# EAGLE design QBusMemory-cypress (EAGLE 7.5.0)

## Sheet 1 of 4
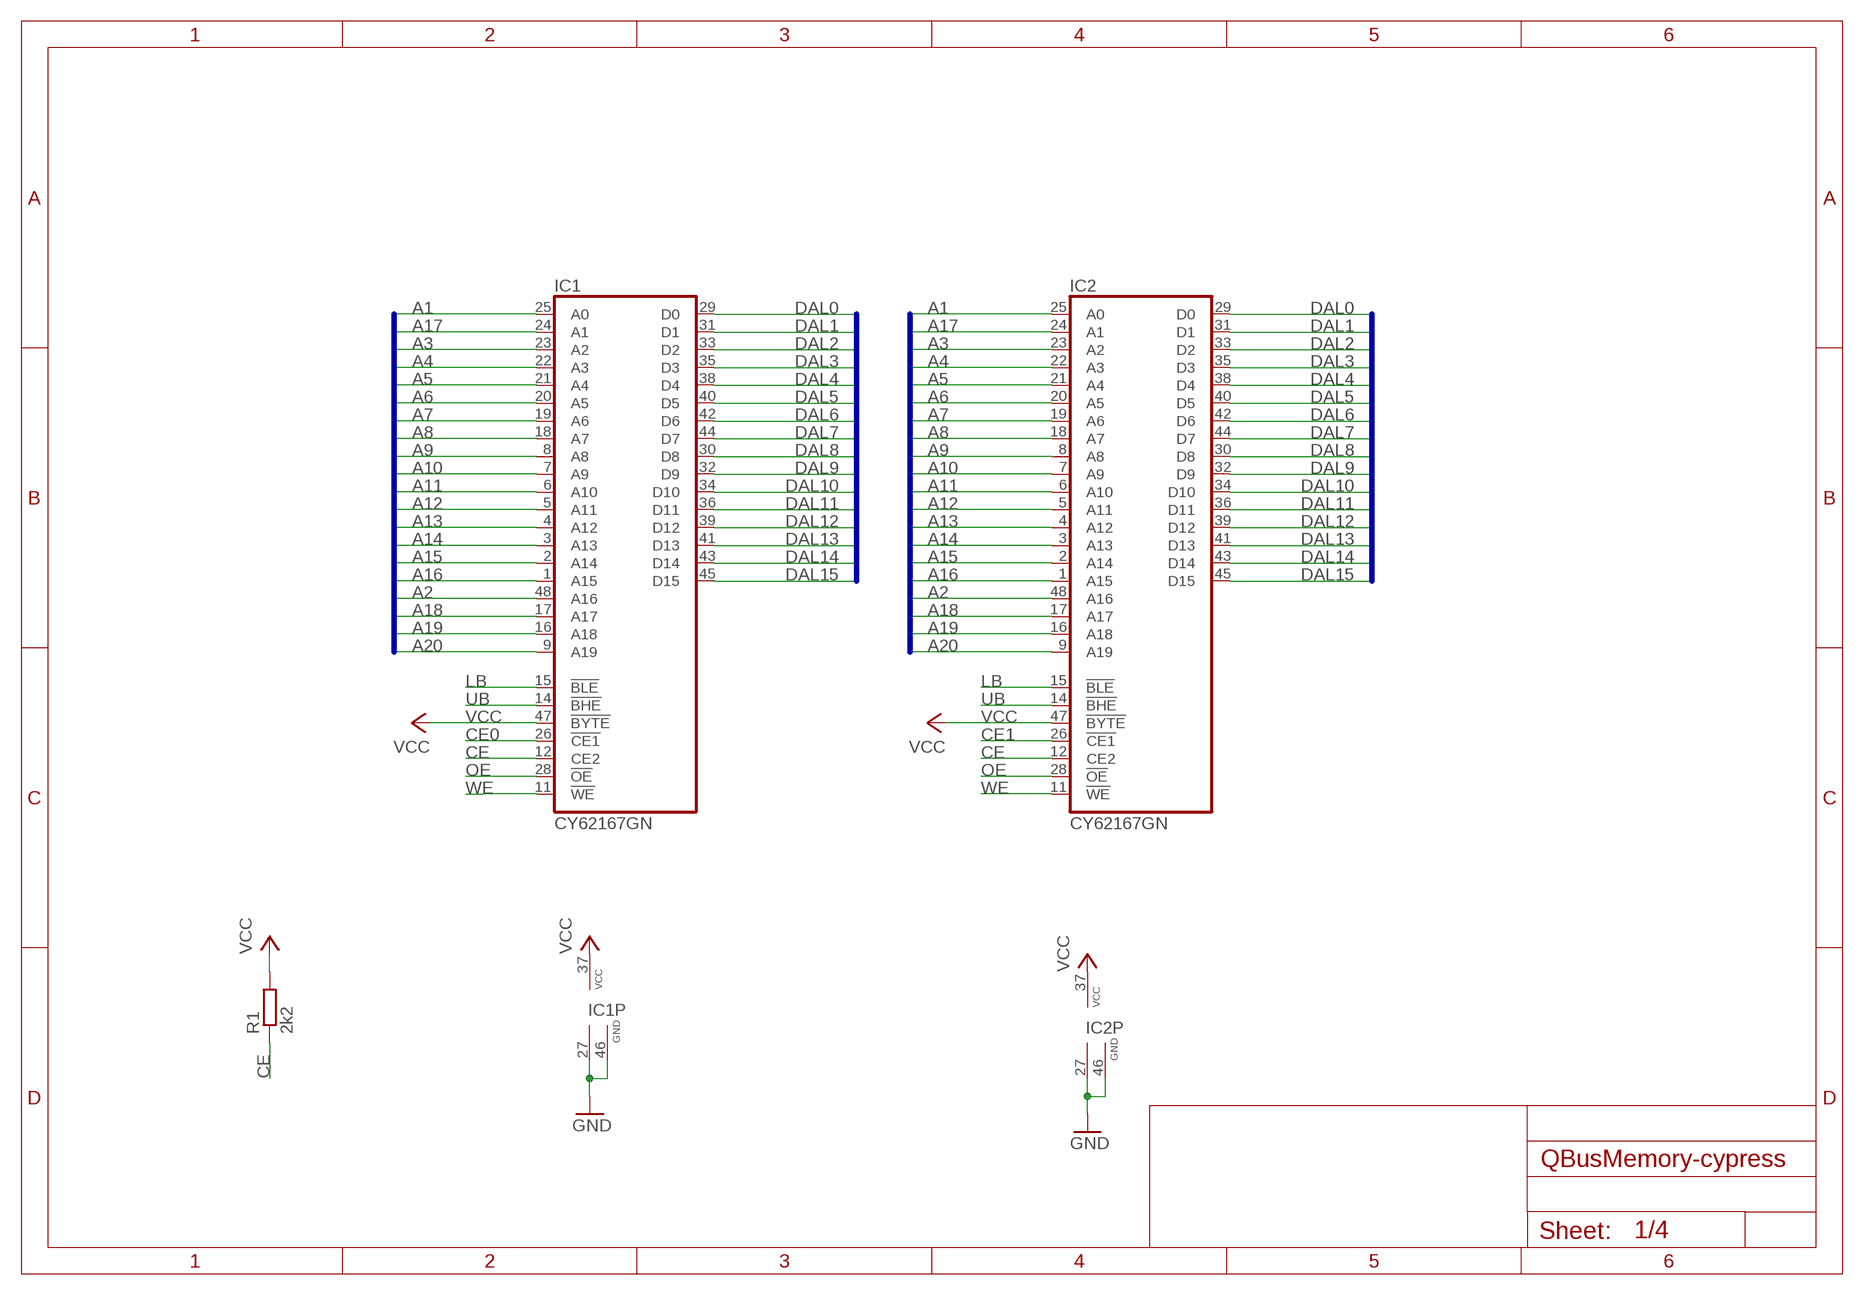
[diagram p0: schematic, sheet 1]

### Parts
IC1  CY62167GN  CY62167  [TSOP48]
IC2  CY62167GN  CY62167  [TSOP48]
R1  2k2  R-EU_R0805  [R0805]

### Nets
A1: IC1.25(A0) IC2.25(A0) ; also sheet 4
A2: IC1.48(A16) IC2.48(A16) ; also sheet 4
A3: IC1.23(A2) IC2.23(A2) ; also sheet 4
A4: IC1.22(A3) IC2.22(A3) ; also sheet 4
A5: IC1.21(A4) IC2.21(A4) ; also sheet 3
A6: IC1.20(A5) IC2.20(A5) ; also sheet 3
A7: IC1.19(A6) IC2.19(A6) ; also sheet 3
A8: IC1.18(A7) IC2.18(A7) ; also sheet 3
A9: IC1.8(A8) IC2.8(A8) ; also sheet 3
A10: IC1.7(A9) IC2.7(A9) ; also sheet 3
A11: IC1.6(A10) IC2.6(A10) ; also sheet 3
A12: IC1.5(A11) IC2.5(A11) ; also sheet 3
A13: IC1.4(A12) IC2.4(A12) ; also sheet 3
A14: IC1.3(A13) IC2.3(A13) ; also sheet 3
A15: IC1.2(A14) IC2.2(A14) ; also sheet 3
A16: IC1.1(A15) IC2.1(A15) ; also sheet 3
A17: IC1.24(A1) IC2.24(A1) ; also sheet 3
A18: IC1.17(A17) IC2.17(A17) ; also sheet 3
A19: IC1.16(A18) IC2.16(A18) ; also sheet 3
A20: IC1.9(A19) IC2.9(A19) ; also sheet 3
CE: IC1.12(CE2) IC2.12(CE2) R1.1
CE0: IC1.26(!CE1) ; also sheet 4
CE1: IC2.26(!CE1) ; also sheet 4
DAL0: IC1.29(D0) IC2.29(D0) ; also sheet 3,4
DAL1: IC1.31(D1) IC2.31(D1) ; also sheet 3,4
DAL2: IC1.33(D2) IC2.33(D2) ; also sheet 3,4
DAL3: IC1.35(D3) IC2.35(D3) ; also sheet 3,4
DAL4: IC1.38(D4) IC2.38(D4) ; also sheet 3,4
DAL5: IC1.40(D5) IC2.40(D5) ; also sheet 3
DAL6: IC1.42(D6) IC2.42(D6) ; also sheet 3
DAL7: IC1.44(D7) IC2.44(D7) ; also sheet 3
DAL8: IC1.30(D8) IC2.30(D8) ; also sheet 3
DAL9: IC1.32(D9) IC2.32(D9) ; also sheet 3
DAL10: IC1.34(D10) IC2.34(D10) ; also sheet 3
DAL11: IC1.36(D11) IC2.36(D11) ; also sheet 3
DAL12: IC1.39(D12) IC2.39(D12) ; also sheet 3
DAL13: IC1.41(D13) IC2.41(D13) ; also sheet 3
DAL14: IC1.43(D14) IC2.43(D14) ; also sheet 3
DAL15: IC1.45(D15) IC2.45(D15) ; also sheet 3
GND: IC1.27(GND) IC1.46(GND) IC2.27(GND) IC2.46(GND) ; also sheet 2,3,4
LB: IC1.15(!BLE) IC2.15(!BLE) ; also sheet 4
OE: IC1.28(!OE) IC2.28(!OE) ; also sheet 4
UB: IC1.14(!BHE) IC2.14(!BHE) ; also sheet 4
VCC: IC1.37(VCC) IC1.47(!BYTE) IC2.37(VCC) IC2.47(!BYTE) R1.2 ; also sheet 2,3,4
WE: IC1.11(!WE) IC2.11(!WE) ; also sheet 4
Unconnected: IC1.10(NC) IC1.13(NC) IC2.10(NC) IC2.13(NC)

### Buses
A[0..21]
DAL[0..21]

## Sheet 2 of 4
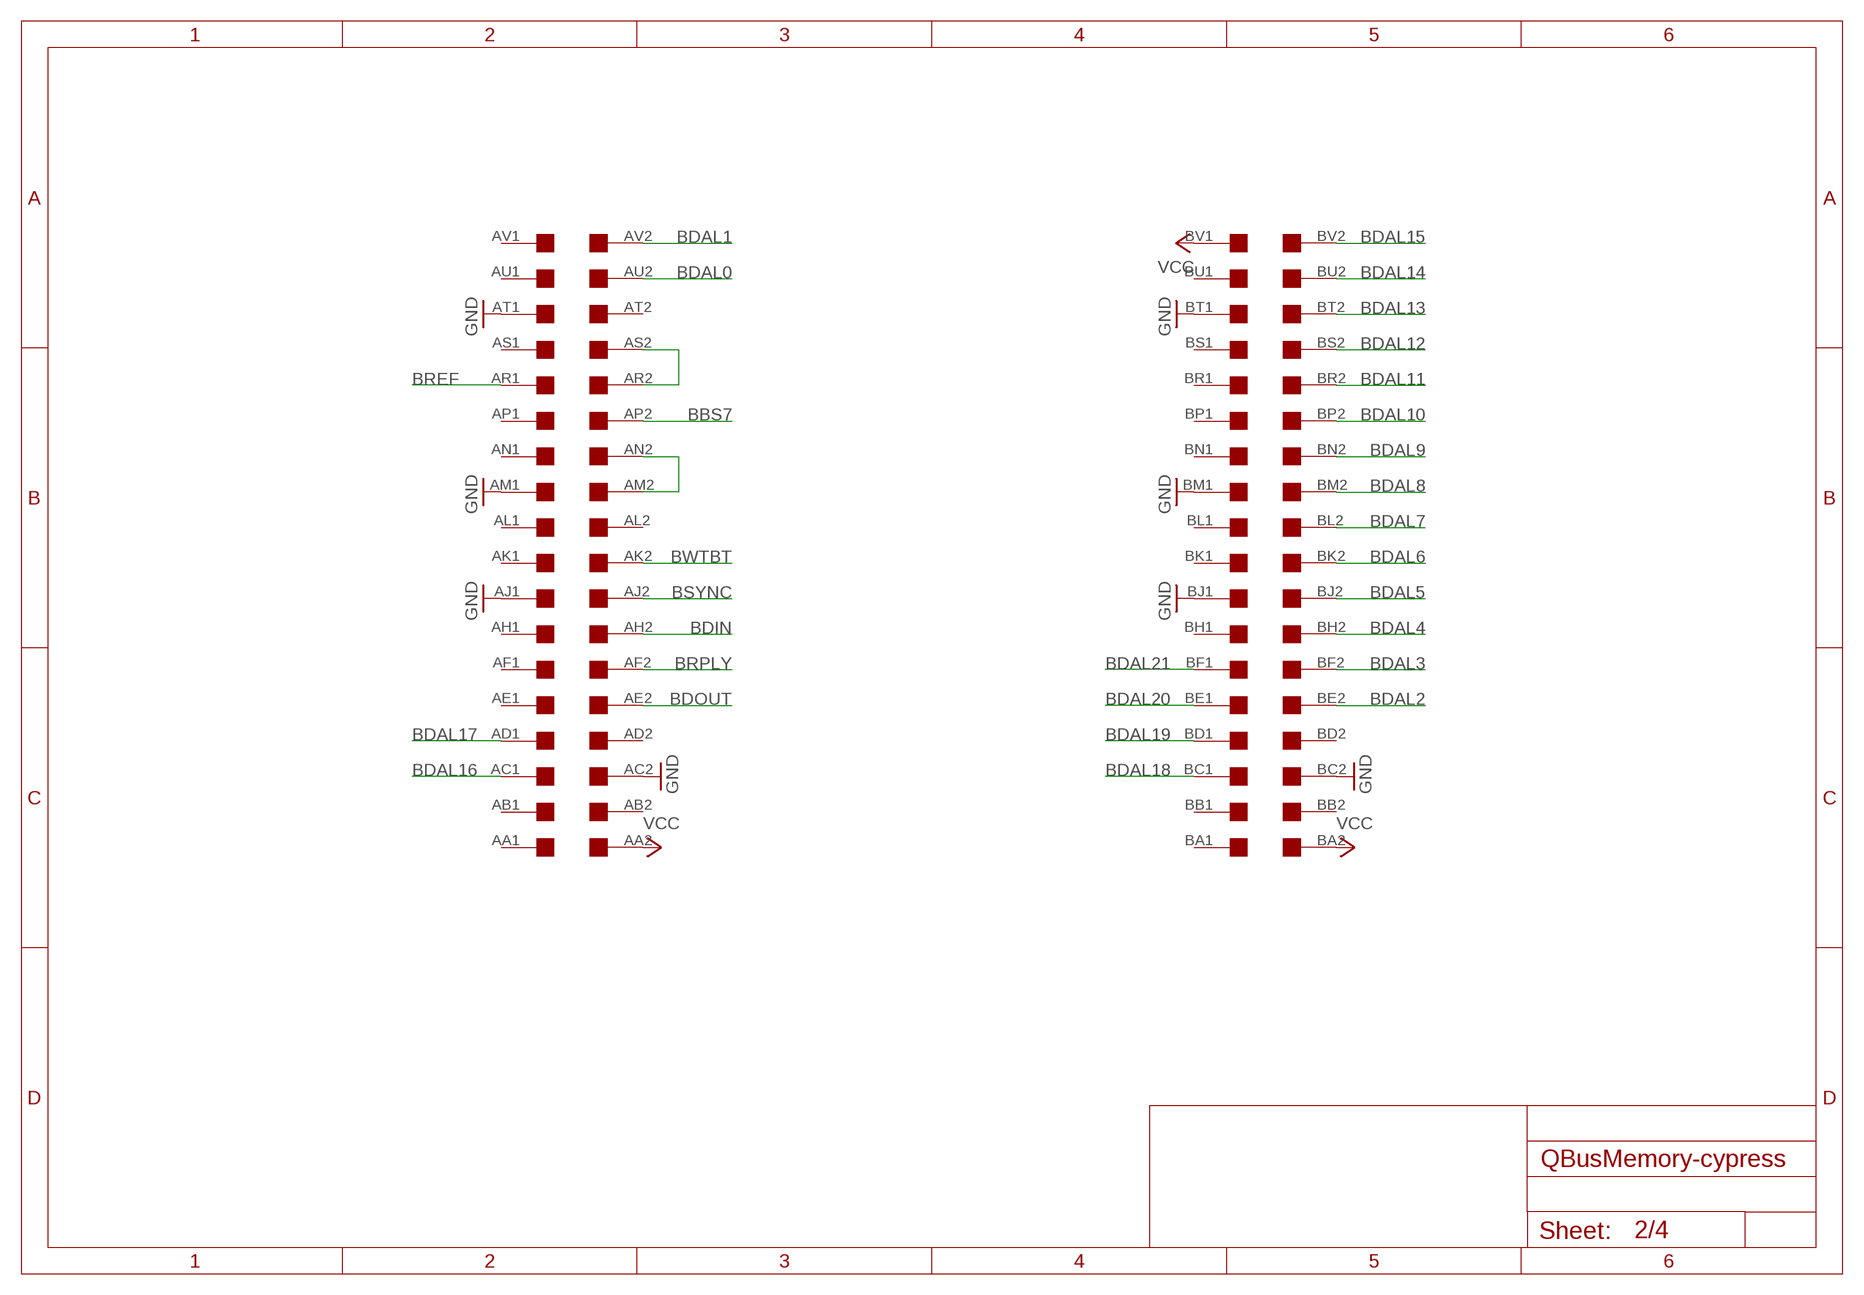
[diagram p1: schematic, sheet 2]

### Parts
U$1  DOUBLE  [EDGE-CON4]

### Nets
BBS7: U$1.AP2 ; also sheet 3
BDAL0: U$1.AU2 ; also sheet 3
BDAL1: U$1.AV2 ; also sheet 3
BDAL2: U$1.BE2 ; also sheet 3
BDAL3: U$1.BF2 ; also sheet 3
BDAL4: U$1.BH2 ; also sheet 3
BDAL5: U$1.BJ2 ; also sheet 3
BDAL6: U$1.BK2 ; also sheet 3
BDAL7: U$1.BL2 ; also sheet 3
BDAL8: U$1.BM2 ; also sheet 3
BDAL9: U$1.BN2 ; also sheet 3
BDAL10: U$1.BP2 ; also sheet 3
BDAL11: U$1.BR2 ; also sheet 3
BDAL12: U$1.BS2 ; also sheet 3
BDAL13: U$1.BT2 ; also sheet 3
BDAL14: U$1.BU2 ; also sheet 3
BDAL15: U$1.BV2 ; also sheet 3
BDAL16: U$1.AC1 ; also sheet 3
BDAL17: U$1.AD1 ; also sheet 3
BDAL18: U$1.BC1 ; also sheet 3
BDAL19: U$1.BD1 ; also sheet 3
BDAL20: U$1.BE1 ; also sheet 3
BDAL21: U$1.BF1 ; also sheet 3
BDIN: U$1.AH2 ; also sheet 3
BDOUT: U$1.AE2 ; also sheet 3
BREF: U$1.AR1 ; also sheet 3
BRPLY: U$1.AF2 ; also sheet 3
BSYNC: U$1.AJ2 ; also sheet 3
BWTBT: U$1.AK2 ; also sheet 3
GND: U$1.AC2 U$1.AJ1 U$1.AM1 U$1.AT1 U$1.BC2 U$1.BJ1 U$1.BM1 U$1.BT1 ; also sheet 1,3,4
N$1: U$1.AR2 U$1.AS2
N$2: U$1.AM2 U$1.AN2
VCC: U$1.AA2 U$1.BA2 U$1.BV1 ; also sheet 1,3,4
Unconnected: U$1.AA1 U$1.AB1 U$1.AB2 U$1.AD2 U$1.AE1 U$1.AF1 U$1.AH1 U$1.AK1 U$1.AL1 U$1.AL2 U$1.AN1 U$1.AP1 U$1.AS1 U$1.AT2 U$1.AU1 U$1.AV1 U$1.BA1 U$1.BB1 U$1.BB2 U$1.BD2 U$1.BH1 U$1.BK1 U$1.BL1 U$1.BN1 U$1.BP1 U$1.BR1 U$1.BS1 U$1.BU1

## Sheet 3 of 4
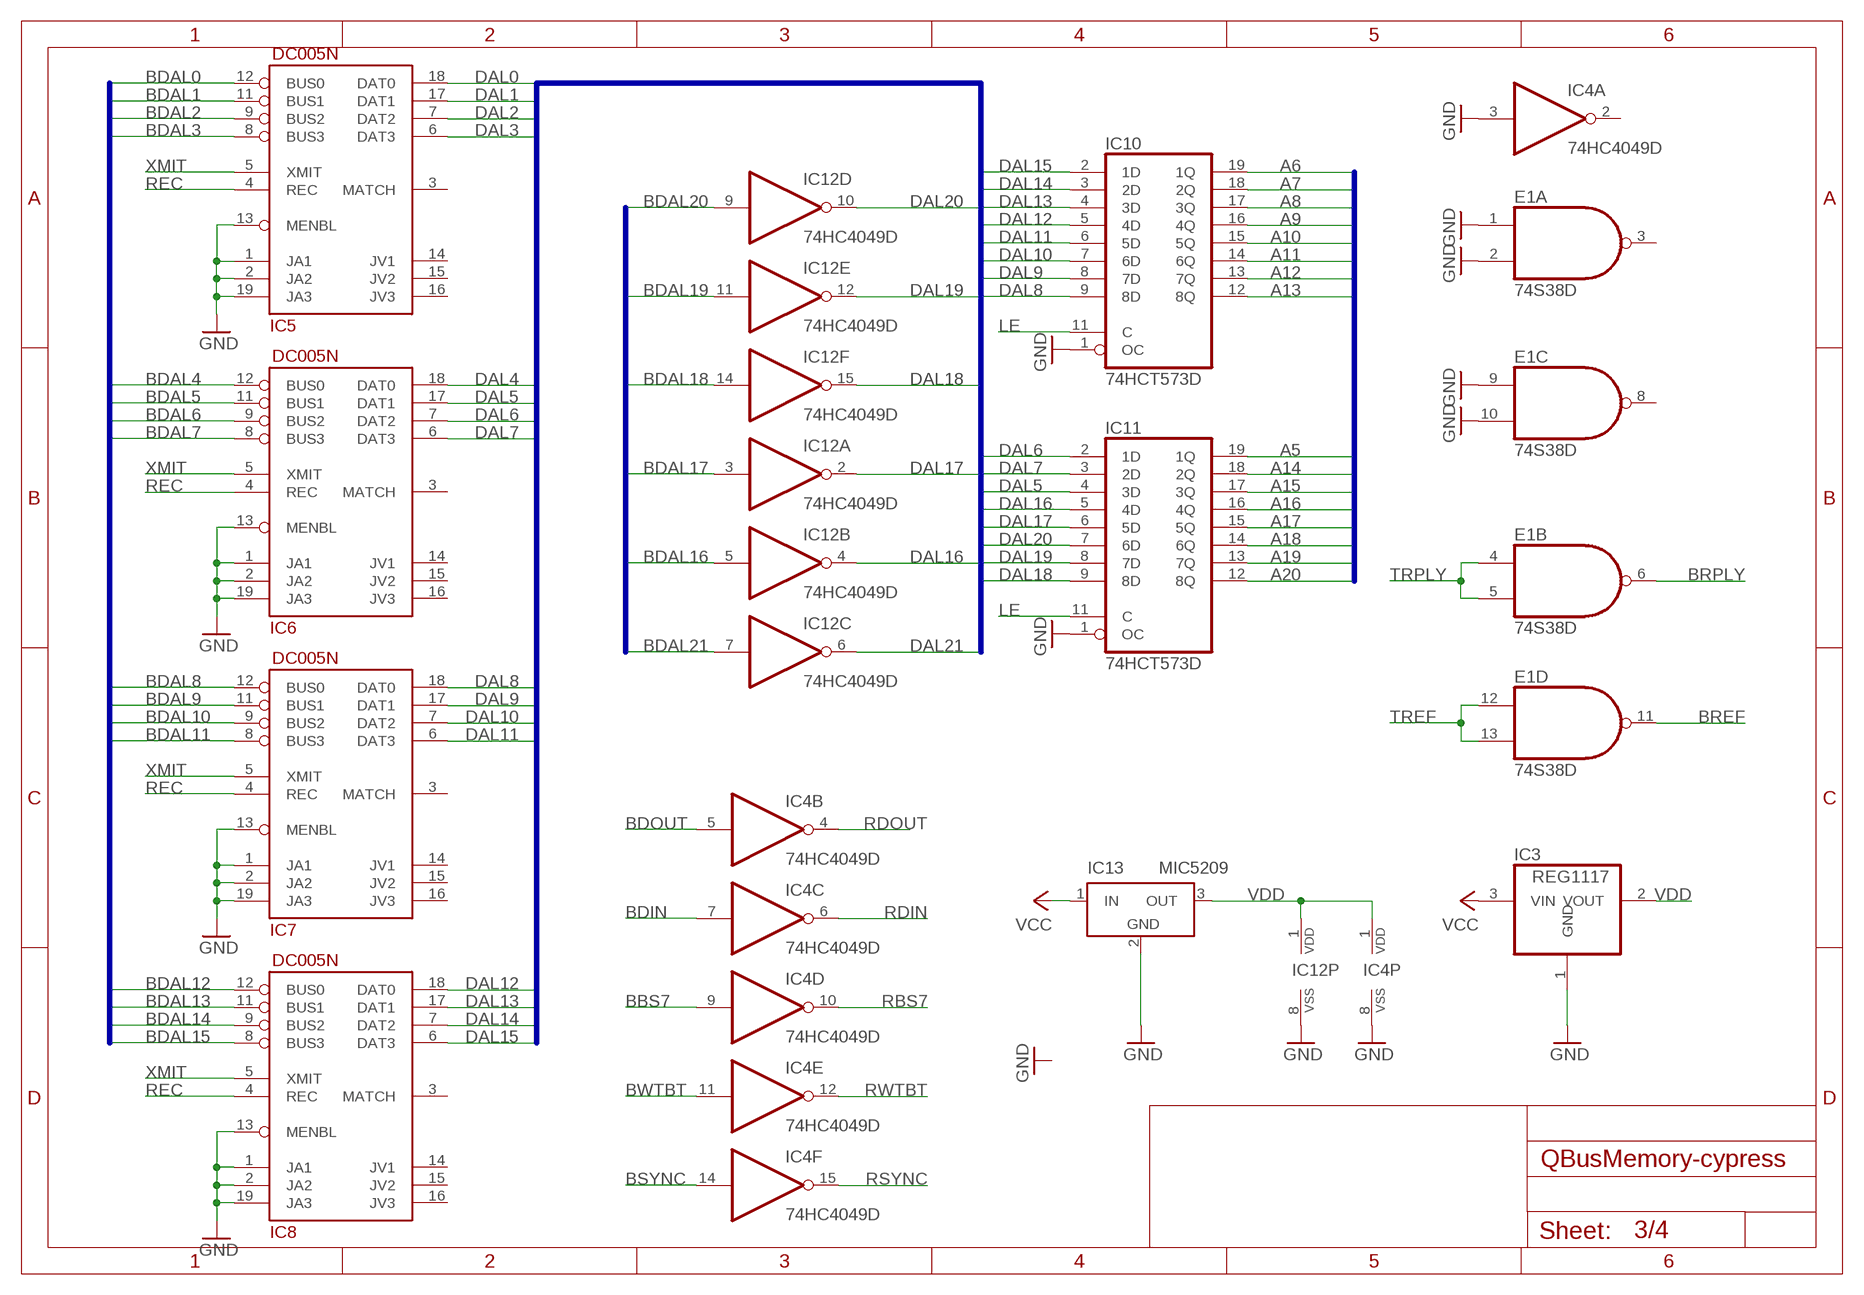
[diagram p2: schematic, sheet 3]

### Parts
E1  74S38D  [SO14]
IC3  REG1117  [SOT223]
IC4  74HC4049D  4049D  [SO16]
IC5  DC005N  [DIL20]
IC6  DC005N  [DIL20]
IC7  DC005N  [DIL20]
IC8  DC005N  [DIL20]
IC10  74HCT573D  [SO20W]
IC11  74HCT573D  [SO20W]
IC12  74HC4049D  4049D  [SO16]
IC13  MIC5209  LT1963EST-3.3  [SOT223]

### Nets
A5: IC11.19(1Q) ; also sheet 1
A6: IC10.19(1Q) ; also sheet 1
A7: IC10.18(2Q) ; also sheet 1
A8: IC10.17(3Q) ; also sheet 1
A9: IC10.16(4Q) ; also sheet 1
A10: IC10.15(5Q) ; also sheet 1
A11: IC10.14(6Q) ; also sheet 1
A12: IC10.13(7Q) ; also sheet 1
A13: IC10.12(8Q) ; also sheet 1
A14: IC11.18(2Q) ; also sheet 1
A15: IC11.17(3Q) ; also sheet 1
A16: IC11.16(4Q) ; also sheet 1
A17: IC11.15(5Q) ; also sheet 1
A18: IC11.14(6Q) ; also sheet 1
A19: IC11.13(7Q) ; also sheet 1
A20: IC11.12(8Q) ; also sheet 1
BBS7: IC4.9(D:I) ; also sheet 2
BDAL0: IC5.12(BUS0) ; also sheet 2
BDAL1: IC5.11(BUS1) ; also sheet 2
BDAL2: IC5.9(BUS2) ; also sheet 2
BDAL3: IC5.8(BUS3) ; also sheet 2
BDAL4: IC6.12(BUS0) ; also sheet 2
BDAL5: IC6.11(BUS1) ; also sheet 2
BDAL6: IC6.9(BUS2) ; also sheet 2
BDAL7: IC6.8(BUS3) ; also sheet 2
BDAL8: IC7.12(BUS0) ; also sheet 2
BDAL9: IC7.11(BUS1) ; also sheet 2
BDAL10: IC7.9(BUS2) ; also sheet 2
BDAL11: IC7.8(BUS3) ; also sheet 2
BDAL12: IC8.12(BUS0) ; also sheet 2
BDAL13: IC8.11(BUS1) ; also sheet 2
BDAL14: IC8.9(BUS2) ; also sheet 2
BDAL15: IC8.8(BUS3) ; also sheet 2
BDAL16: IC12.5(B:I) ; also sheet 2
BDAL17: IC12.3(A:I) ; also sheet 2
BDAL18: IC12.14(F:I) ; also sheet 2
BDAL19: IC12.11(E:I) ; also sheet 2
BDAL20: IC12.9(D:I) ; also sheet 2
BDAL21: IC12.7(C:I) ; also sheet 2
BDIN: IC4.7(C:I) ; also sheet 2
BDOUT: IC4.5(B:I) ; also sheet 2
BREF: E1.11(D:O) ; also sheet 2
BRPLY: E1.6(B:O) ; also sheet 2
BSYNC: IC4.14(F:I) ; also sheet 2
BWTBT: IC4.11(E:I) ; also sheet 2
DAL0: IC5.18(DAT0) ; also sheet 1,4
DAL1: IC5.17(DAT1) ; also sheet 1,4
DAL2: IC5.7(DAT2) ; also sheet 1,4
DAL3: IC5.6(DAT3) ; also sheet 1,4
DAL4: IC6.18(DAT0) ; also sheet 1,4
DAL5: IC6.17(DAT1) IC11.4(3D) ; also sheet 1
DAL6: IC6.7(DAT2) IC11.2(1D) ; also sheet 1
DAL7: IC6.6(DAT3) IC11.3(2D) ; also sheet 1
DAL8: IC7.18(DAT0) IC10.9(8D) ; also sheet 1
DAL9: IC7.17(DAT1) IC10.8(7D) ; also sheet 1
DAL10: IC7.7(DAT2) IC10.7(6D) ; also sheet 1
DAL11: IC7.6(DAT3) IC10.6(5D) ; also sheet 1
DAL12: IC8.18(DAT0) IC10.5(4D) ; also sheet 1
DAL13: IC8.17(DAT1) IC10.4(3D) ; also sheet 1
DAL14: IC8.7(DAT2) IC10.3(2D) ; also sheet 1
DAL15: IC8.6(DAT3) IC10.2(1D) ; also sheet 1
DAL16: IC11.5(4D) IC12.4(B:O)
DAL17: IC11.6(5D) IC12.2(A:O)
DAL18: IC11.9(8D) IC12.15(F:O)
DAL19: IC11.8(7D) IC12.12(E:O)
DAL20: IC11.7(6D) IC12.10(D:O)
DAL21: IC12.6(C:O) ; also sheet 4
GND: E1.1(A:I0) E1.2(A:I1) E1.9(C:I0) E1.10(C:I1) IC3.1(GND) IC4.3(A:I) IC4.8(P:VSS) IC5.1(JA1) IC5.2(JA2) IC5.13(MENBL) IC5.19(JA3) IC6.1(JA1) IC6.2(JA2) IC6.13(MENBL) IC6.19(JA3) IC7.1(JA1) IC7.2(JA2) IC7.13(MENBL) IC7.19(JA3) IC8.1(JA1) IC8.2(JA2) IC8.13(MENBL) IC8.19(JA3) IC10.1(OC) IC11.1(OC) IC12.8(P:VSS) IC13.2(GND) ; also sheet 1,2,4
LE: IC10.11(C) IC11.11(C) ; also sheet 4
RBS7: IC4.10(D:O) ; also sheet 4
RDIN: IC4.6(C:O) ; also sheet 4
RDOUT: IC4.4(B:O) ; also sheet 4
REC: IC5.4(REC) IC6.4(REC) IC7.4(REC) IC8.4(REC) ; also sheet 4
RSYNC: IC4.15(F:O) ; also sheet 4
RWTBT: IC4.12(E:O) ; also sheet 4
TREF: E1.12(D:I0) E1.13(D:I1) ; also sheet 4
TRPLY: E1.4(B:I0) E1.5(B:I1) ; also sheet 4
VCC: IC3.3(VIN) IC13.1(IN) ; also sheet 1,2,4
VDD: IC3.2(VOUT) IC4.1(P:VDD) IC12.1(P:VDD) IC13.3(OUT) ; also sheet 4
XMIT: IC5.5(XMIT) IC6.5(XMIT) IC7.5(XMIT) IC8.5(XMIT) ; also sheet 4
Unconnected: E1.3(A:O) E1.8(C:O) IC4.2(A:O) IC5.3(MATCH) IC5.14(JV1) IC5.15(JV2) IC5.16(JV3) IC6.3(MATCH) IC6.14(JV1) IC6.15(JV2) IC6.16(JV3) IC7.3(MATCH) IC7.14(JV1) IC7.15(JV2) IC7.16(JV3) IC8.3(MATCH) IC8.14(JV1) IC8.15(JV2) IC8.16(JV3)

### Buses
DAL[0..21]
BDAL[0..21]
A[0..21]

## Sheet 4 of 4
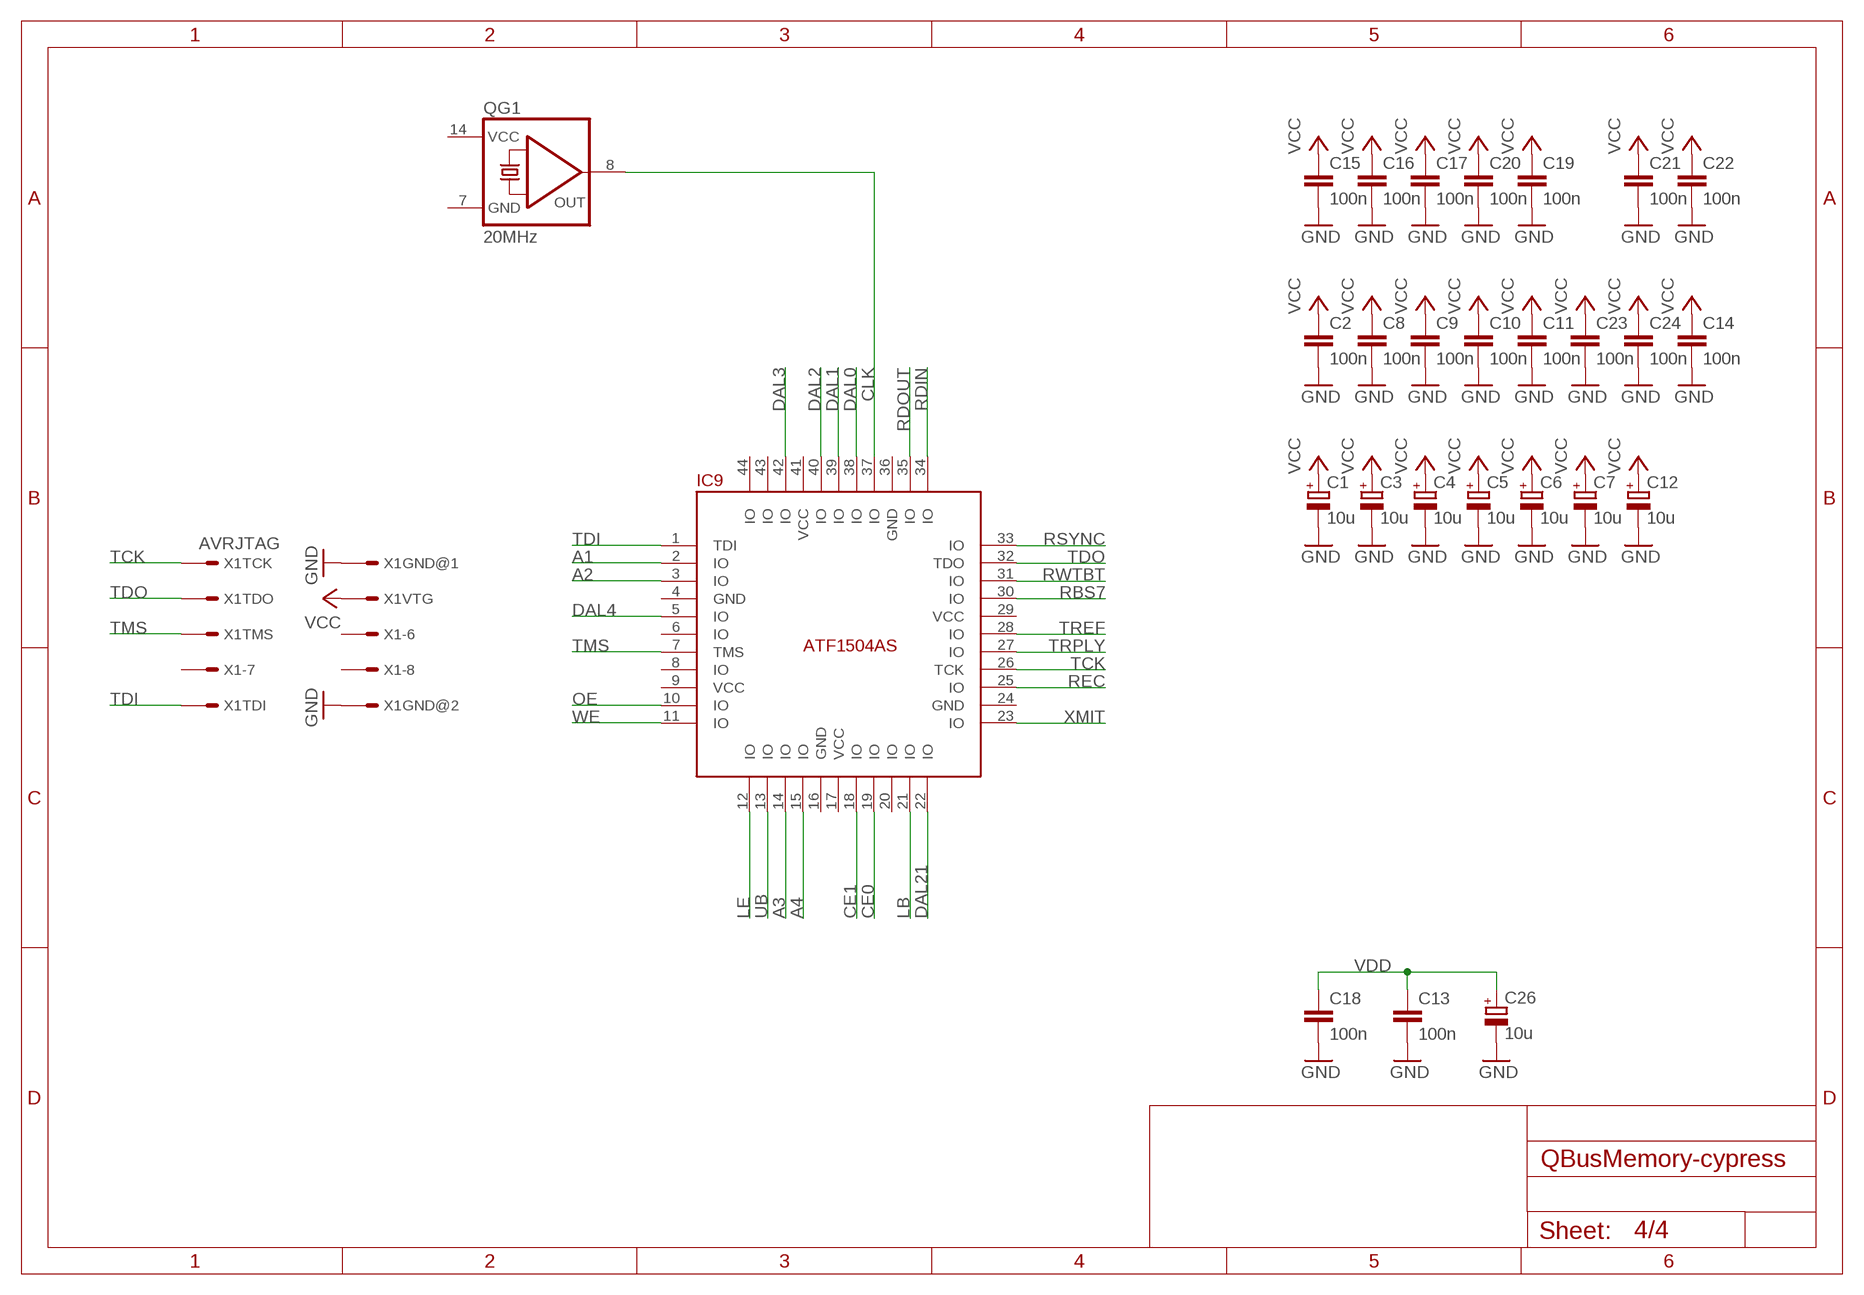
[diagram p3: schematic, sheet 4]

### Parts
C1  10u  CPOL-EUSMCC  [SMC_C]
C2  100n  C-EUC0805  [C0805]
C3  10u  CPOL-EUSMCC  [SMC_C]
C4  10u  CPOL-EUSMCC  [SMC_C]
C5  10u  CPOL-EUSMCC  [SMC_C]
C6  10u  CPOL-EUSMCC  [SMC_C]
C7  10u  CPOL-EUSMCC  [SMC_C]
C8  100n  C-EUC0805  [C0805]
C9  100n  C-EUC0805  [C0805]
C10  100n  C-EUC0805  [C0805]
C11  100n  C-EUC0805  [C0805]
C12  10u  CPOL-EUSMCC  [SMC_C]
C13  100n  C-EUC0805  [C0805]
C14  100n  C-EUC0805  [C0805]
C15  100n  C-EUC0805  [C0805]
C16  100n  C-EUC0805  [C0805]
C17  100n  C-EUC0805  [C0805]
C18  100n  C-EUC0805  [C0805]
C19  100n  C-EUC0805  [C0805]
C20  100n  C-EUC0805  [C0805]
C21  100n  C-EUC0805  [C0805]
C22  100n  C-EUC0805  [C0805]
C23  100n  C-EUC0805  [C0805]
C24  100n  C-EUC0805  [C0805]
C26  10u  CPOL-EUSMCC  [SMC_C]
IC9  ATF1504AS  [TQFP44]
QG1  20MHz  QG5860  [DIL14S]
X1  AVRJTAG  [ML10L]

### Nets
A1: IC9.2(IO) ; also sheet 1
A2: IC9.3(IO) ; also sheet 1
A3: IC9.14(IO) ; also sheet 1
A4: IC9.15(IO) ; also sheet 1
CE0: IC9.19(IO) ; also sheet 1
CE1: IC9.18(IO) ; also sheet 1
CLK: IC9.37(IO) QG1.8(OUT)
DAL0: IC9.38(IO) ; also sheet 1,3
DAL1: IC9.39(IO) ; also sheet 1,3
DAL2: IC9.40(IO) ; also sheet 1,3
DAL3: IC9.42(IO) ; also sheet 1,3
DAL4: IC9.5(IO) ; also sheet 1,3
DAL21: IC9.22(IO) ; also sheet 3
GND: C1.- C2.2 C3.- C4.- C5.- C6.- C7.- C8.2 C9.2 C10.2 C11.2 C12.- C13.2 C14.2 C15.2 C16.2 C17.2 C18.2 C19.2 C20.2 C21.2 C22.2 C23.2 C24.2 C26.- X1.2 X1.10 ; also sheet 1,2,3
LB: IC9.21(IO) ; also sheet 1
LE: IC9.12(IO) ; also sheet 3
OE: IC9.10(IO) ; also sheet 1
RBS7: IC9.30(IO) ; also sheet 3
RDIN: IC9.34(IO) ; also sheet 3
RDOUT: IC9.35(IO) ; also sheet 3
REC: IC9.25(IO) ; also sheet 3
RSYNC: IC9.33(IO) ; also sheet 3
RWTBT: IC9.31(IO) ; also sheet 3
TCK: IC9.26(TCK) X1.1
TDI: IC9.1(TDI) X1.9
TDO: IC9.32(TDO) X1.3
TMS: IC9.7(TMS) X1.5
TREF: IC9.28(IO) ; also sheet 3
TRPLY: IC9.27(IO) ; also sheet 3
UB: IC9.13(IO) ; also sheet 1
VCC: C1.+ C2.1 C3.+ C4.+ C5.+ C6.+ C7.+ C8.1 C9.1 C10.1 C11.1 C12.+ C14.1 C15.1 C16.1 C17.1 C19.1 C20.1 C21.1 C22.1 C23.1 C24.1 X1.4 ; also sheet 1,2,3
VDD: C13.1 C18.1 C26.+ ; also sheet 3
WE: IC9.11(IO) ; also sheet 1
XMIT: IC9.23(IO) ; also sheet 3
Unconnected: IC9.6(IO) IC9.8(IO) IC9.20(IO) IC9.43(IO) IC9.44(IO) X1.6 X1.7 X1.8

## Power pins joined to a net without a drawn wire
GND: E1.7(P:GND) IC5.10(GND) IC6.10(GND) IC7.10(GND) IC8.10(GND) IC9.4(GND) IC9.16(GND) IC9.24(GND) IC9.36(GND) IC10.10(GND) IC11.10(GND) IC13.4(GND) QG1.7(GND)
VCC: E1.14(P:VCC) IC5.20(VCC) IC6.20(VCC) IC7.20(VCC) IC8.20(VCC) IC9.9(VCC) IC9.17(VCC) IC9.29(VCC) IC9.41(VCC) IC10.20(VCC) IC11.20(VCC) QG1.14(VCC)

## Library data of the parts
C1 C3-C7 C12 C26 = rcl:CPOL-EU: POLARIZED CAPACITOR, European symbol
C2 C8-C11 C13-C24 = rcl:C-EU: CAPACITOR, European symbol
E1 = dec-con:74*38: Quad 2-input NAND gate, open collector output
IC1 IC2 = cbscpe_eagle60:CY62167: 4-Megabit FLASH MEMORY (512 K x 8 bit/256 K x 16 bit CMOS 3 V-only boot sector flash memory
IC3 = burr-brown:REG1117: 800mA and 1A Low Dropout (LDO) Positive Regulator 1.8V, 2.5V, 2.85V, 3.3V, 5V, and Adj; MPN: REG1117; OC_FARNELL: 1097566; OC_NEWARK: 14P6981
IC4 IC12 = 40xx:4049: Hex inverting BUFFER
IC5-IC8 = cbscpe_eagle60:DC005
IC9 = cbscpe_eagle60:ATF1504AS: Generic ATF1504AS
IC10 IC11 = 74xx-eu:74*573: 8-bit D latch BUS DRIVER
IC13 = linear-technology:LT1963EST: 1.5A, Low Noise, Fast Transient Response LDO Regulator Source: http://www.linear.com/pc/downloadDocument.do?navId=H0,C3,P2222,D3148; MPN: LT1963EST-3.3; OC_FARNELL: 1501032; OC_NEWARK: 57M7546
QG1 = crystal:QG5860: CRYSTAL RESONATOR; OC_FARNELL: unknown; OC_NEWARK: unknown
R1 = rcl:R-EU_: RESISTOR, European symbol
U$1 = dec-con:DOUBLE: Double-Height DEC board
X1 = cbscpe_eagle60:AVRJTAG: CONNECTOR 10-pin series 057 contact pc board low profile headers

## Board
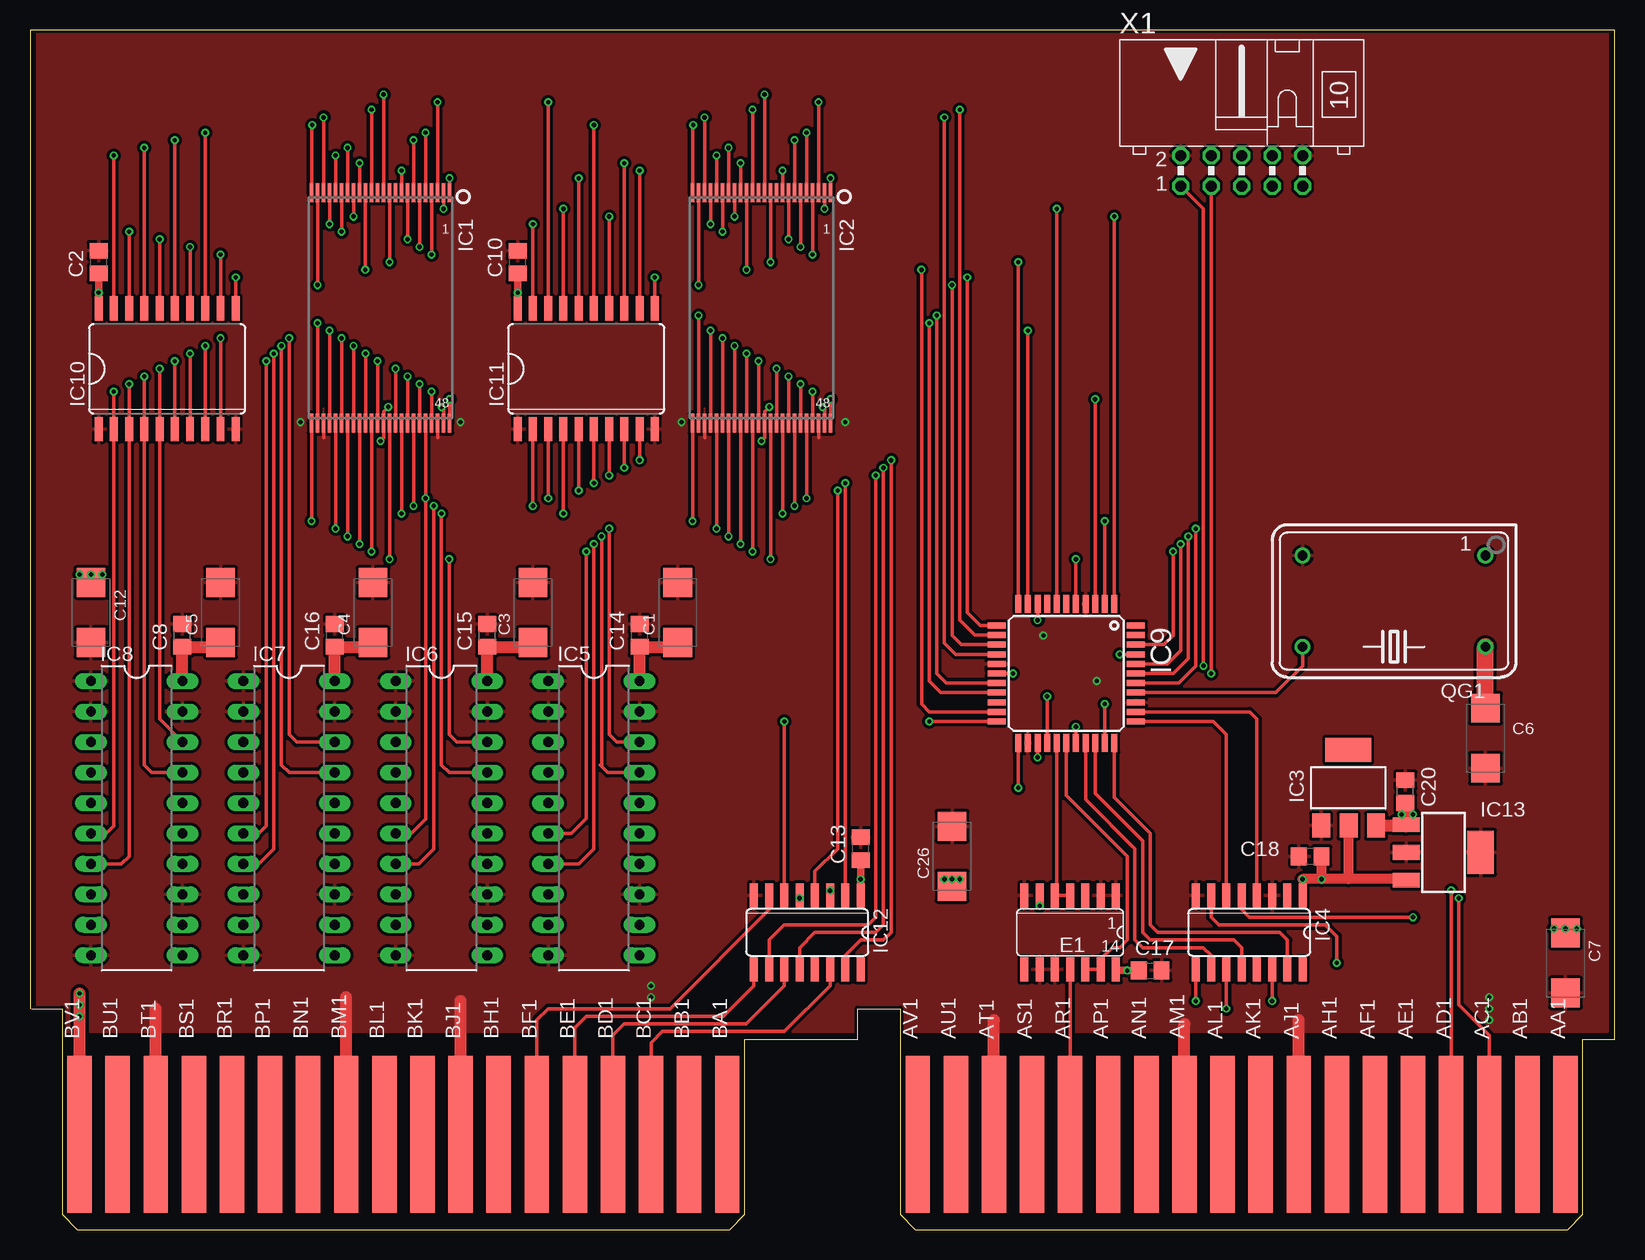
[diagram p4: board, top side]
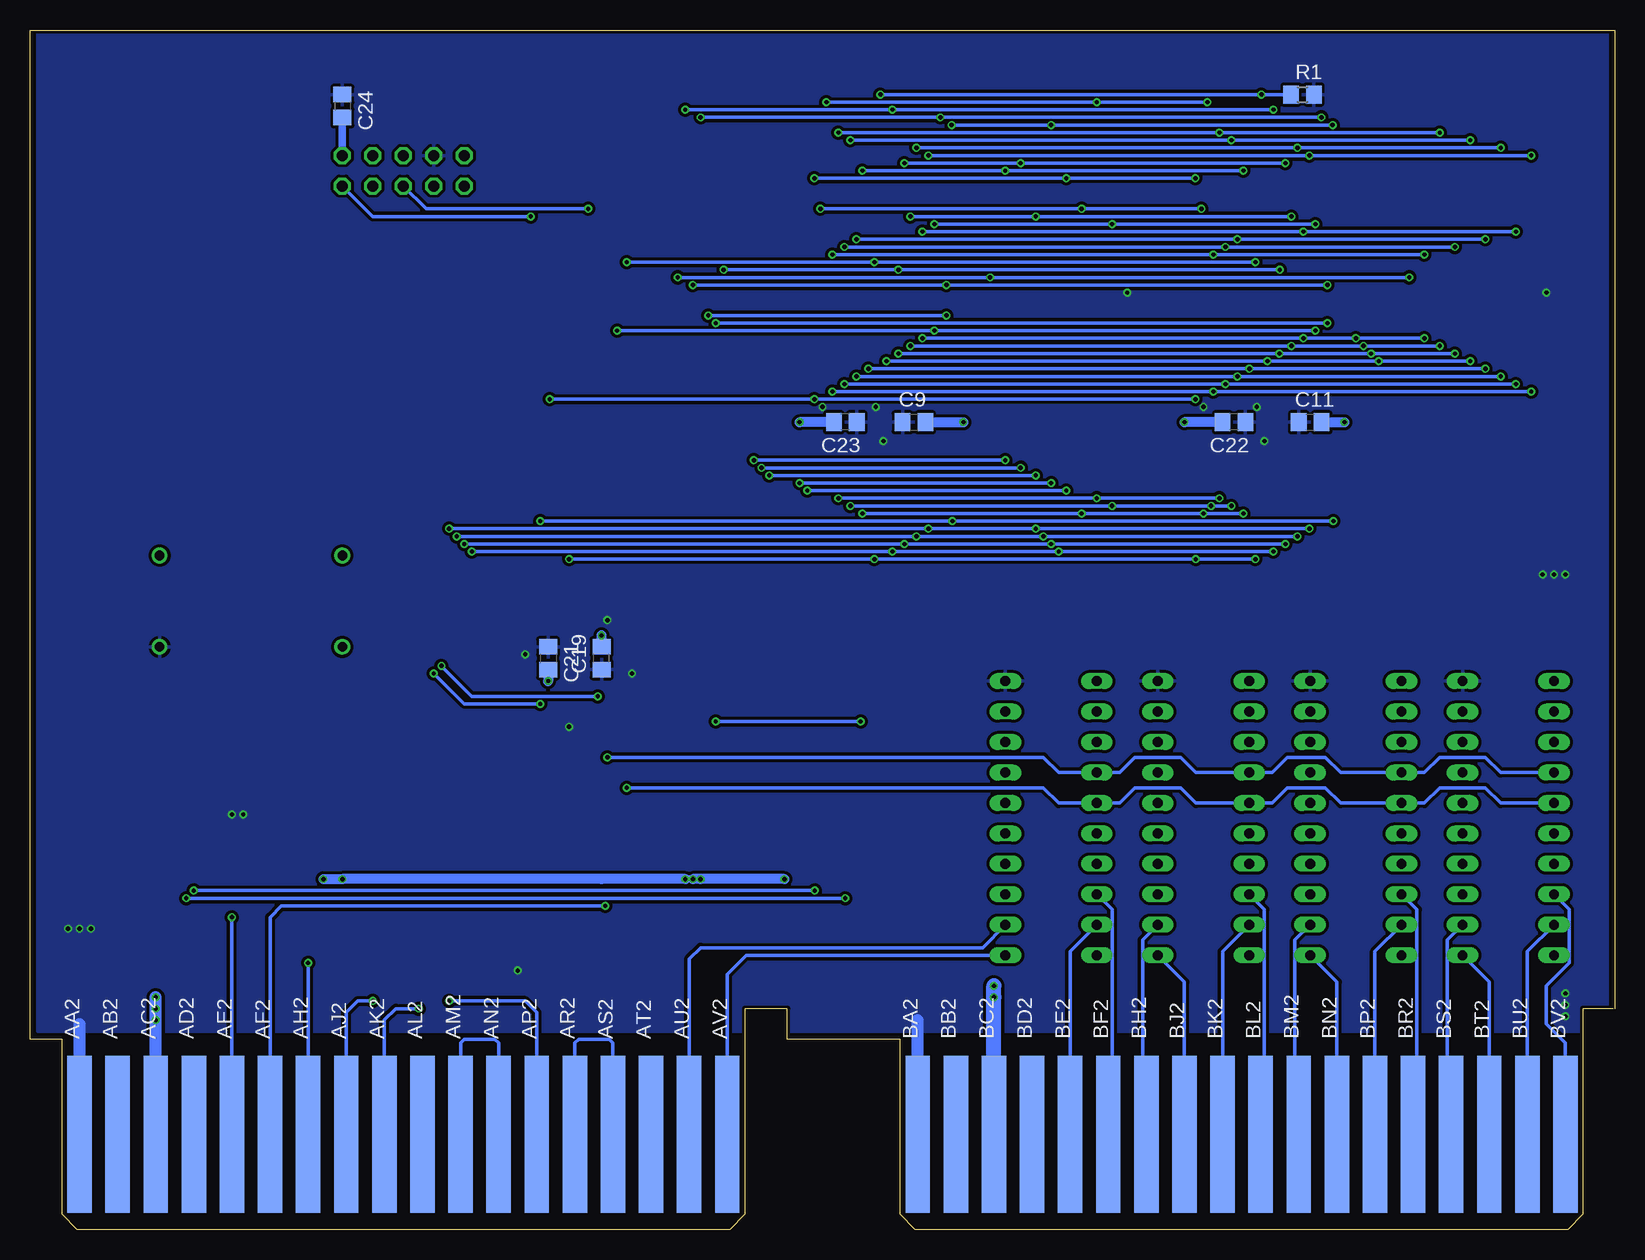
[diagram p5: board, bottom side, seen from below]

Size 132.08 x 100 mm. Coordinates in mm from the lower left corner, seen from the top.
Outline: 132.06,15.88 132.06,100 0,100 0,18.41
Copper layers (1*16): Top 0.035mm / dielectric 1.5mm / Bottom 0.035mm
Design rules "dirt_cheap_dirty_boards.v1a *": minimum track width 5mil, minimum drill 12mil, track to track 5mil, track to pad 5mil, pad to pad 5mil, via to via 5mil, smd to smd 0mil, copper to edge 10mil, drill to drill 10mil, minimum pad ring 10mil, minimum via ring 6mil, stop-mask expansion 2mil, vias tented up to drill 25mil, thermal gap 10mil

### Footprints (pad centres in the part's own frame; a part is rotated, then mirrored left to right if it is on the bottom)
SMC_C = smd 2.4 x 2.4: + -2.5,0; - 2.5,0
C0805 = smd 1.3 x 1.5: 1 -0.95,0; 2 0.95,0
SO14 = smd 0.66 x 2.032: 1 -3.81,-3.073; 2 -2.54,-3.073; 3 -1.27,-3.073; 4 0,-3.073; 5 1.27,-3.073; 6 2.54,-3.073; 7 3.81,-3.073; 8 3.81,3.073; 9 2.54,3.073; 10 1.27,3.073; 11 0,3.073; 12 -1.27,3.073; 13 -2.54,3.073; 14 -3.81,3.073
TSOP48 = smd 0.3 x 1.6: 1 -5.75,-9.6; 2 -5.25,-9.6; 3 -4.75,-9.6; 4 -4.25,-9.6; 5 -3.75,-9.6; 6 -3.25,-9.6; 7 -2.75,-9.6; 8 -2.25,-9.6; 9 -1.75,-9.6; 10 -1.25,-9.6; 11 -0.75,-9.6; 12 -0.25,-9.6; 13 0.25,-9.6; 14 0.75,-9.6; 15 1.25,-9.6; 16 1.75,-9.6; 17 2.25,-9.6; 18 2.75,-9.6; 19 3.25,-9.6; 20 3.75,-9.6; 21 4.25,-9.6; 22 4.75,-9.6; 23 5.25,-9.6; 24 5.75,-9.6; 25 5.75,9.6; 26 5.25,9.6; 27 4.75,9.6; 28 4.25,9.6; 29 3.75,9.6; 30 3.25,9.6; 31 2.75,9.6; 32 2.25,9.6; 33 1.75,9.6; 34 1.25,9.6; 35 0.75,9.6; 36 0.25,9.6; 37 -0.25,9.6; 38 -0.75,9.6; 39 -1.25,9.6; 40 -1.75,9.6; 41 -2.25,9.6; 42 -2.75,9.6; 43 -3.25,9.6; 44 -3.75,9.6; 45 -4.25,9.6; 46 -4.75,9.6; 47 -5.25,9.6; 48 -5.75,9.6
SOT223 = smd 1.499 x 2.007: 1 -2.261,-3.15; 2 0.025,-3.15; 3 2.311,-3.15 | smd 3.81 x 2.007: 4 0,3.15
SO16 = smd 0.66 x 2.032: 1 -4.445,-3.073; 2 -3.175,-3.073; 3 -1.905,-3.073; 4 -0.635,-3.073; 5 0.635,-3.073; 6 1.905,-3.073; 7 3.175,-3.073; 8 4.445,-3.073; 9 4.445,3.073; 10 3.175,3.073; 11 1.905,3.073; 12 0.635,3.073; 13 -0.635,3.073; 14 -1.905,3.073; 15 -3.175,3.073; 16 -4.445,3.073
DIL20 = drill 0.813 long: 1 -11.43,-3.81; 2 -8.89,-3.81; 3 -6.35,-3.81; 4 -3.81,-3.81; 5 -1.27,-3.81; 6 1.27,-3.81; 7 3.81,-3.81; 8 6.35,-3.81; 9 8.89,-3.81; 10 11.43,-3.81; 11 11.43,3.81; 12 8.89,3.81; 13 6.35,3.81; 14 3.81,3.81; 15 1.27,3.81; 16 -1.27,3.81; 17 -3.81,3.81; 18 -6.35,3.81; 19 -8.89,3.81; 20 -11.43,3.81
TQFP44 = smd 1.5 x 0.5: 1 -5.8,4; 2 -5.8,3.2; 3 -5.8,2.4; 4 -5.8,1.6; 5 -5.8,0.8; 6 -5.8,0; 7 -5.8,-0.8; 8 -5.8,-1.6; 9 -5.8,-2.4; 10 -5.8,-3.2; 11 -5.8,-4; 23 5.8,-4; 24 5.8,-3.2; 25 5.8,-2.4; 26 5.8,-1.6; 27 5.8,-0.8; 28 5.8,0; 29 5.8,0.8; 30 5.8,1.6; 31 5.8,2.4; 32 5.8,3.2; 33 5.8,4 | smd 0.5 x 1.5: 12 -4,-5.8; 13 -3.2,-5.8; 14 -2.4,-5.8; 15 -1.6,-5.8; 16 -0.8,-5.8; 17 0,-5.8; 18 0.8,-5.8; 19 1.6,-5.8; 20 2.4,-5.8; 21 3.2,-5.8; 22 4,-5.8; 34 4,5.8; 35 3.2,5.8; 36 2.4,5.8; 37 1.6,5.8; 38 0.8,5.8; 39 0,5.8; 40 -0.8,5.8; 41 -1.6,5.8; 42 -2.4,5.8; 43 -3.2,5.8; 44 -4,5.8
SO20W = smd 0.66 x 2.032: 1 -5.715,-5.029; 2 -4.445,-5.029; 3 -3.175,-5.029; 4 -1.905,-5.029; 5 -0.635,-5.029; 6 0.635,-5.029; 7 1.905,-5.029; 8 3.175,-5.029; 9 4.445,-5.029; 10 5.715,-5.029; 11 5.715,5.029; 12 4.445,5.029; 13 3.175,5.029; 14 1.905,5.029; 15 0.635,5.029; 16 -0.635,5.029; 17 -1.905,5.029; 18 -3.175,5.029; 19 -4.445,5.029; 20 -5.715,5.029
SOT223' = smd 1.219 x 2.235: 1 -2.311,-3.099; 2 0,-3.099; 3 2.311,-3.099 | smd 3.6 x 2.2: 4 0,3.099
DIL14S = drill 0.813: 1 -7.62,-3.81; 7 7.62,-3.81; 8 7.62,3.81; 14 -7.62,3.81
R0805 = smd 1.3 x 1.5: 1 -0.95,0; 2 0.95,0
EDGE-CON4 = smd 13.106 x 2.032: AA1 7.938,4.128; AB1 7.938,7.303; AC1 7.938,10.477; AD1 7.938,13.652; AE1 7.938,16.828; AF1 7.938,20.003; AH1 7.938,23.177; AJ1 7.938,26.352; AK1 7.938,29.527; AL1 7.938,32.703; AM1 7.938,35.877; AN1 7.938,39.053; AP1 7.938,42.227; AR1 7.938,45.403; AS1 7.938,48.578; AT1 7.938,51.752; AU1 7.938,54.928; AV1 7.938,58.102; BA1 7.938,73.978; BB1 7.938,77.153; BC1 7.938,80.328; BD1 7.938,83.502; BE1 7.938,86.677; BF1 7.938,89.853; BH1 7.938,93.028; BJ1 7.938,96.203; BK1 7.938,99.377; BL1 7.938,102.552; BM1 7.938,105.728; BN1 7.938,108.903; BP1 7.938,112.078; BR1 7.938,115.252; BS1 7.938,118.427; BT1 7.938,121.603; BU1 7.938,124.778; BV1 7.938,127.953 | smd 13.106 x 2.032 bottom: AA2 7.938,4.128; AB2 7.938,7.303; AC2 7.938,10.477; AD2 7.938,13.652; AE2 7.938,16.828; AF2 7.938,20.003; AH2 7.938,23.177; AJ2 7.938,26.352; AK2 7.938,29.527; AL2 7.938,32.703; AM2 7.938,35.877; AN2 7.938,39.053; AP2 7.938,42.227; AR2 7.938,45.403; AS2 7.938,48.578; AT2 7.938,51.752; AU2 7.938,54.928; AV2 7.938,58.102; BA2 7.938,73.978; BB2 7.938,77.153; BC2 7.938,80.328; BD2 7.938,83.502; BE2 7.938,86.677; BF2 7.938,89.853; BH2 7.938,93.028; BJ2 7.938,96.203; BK2 7.938,99.377; BL2 7.938,102.552; BM2 7.938,105.728; BN2 7.938,108.903; BP2 7.938,112.078; BR2 7.938,115.252; BS2 7.938,118.427; BT2 7.938,121.603; BU2 7.938,124.778; BV2 7.938,127.953
ML10L = drill 0.914 octagon: 1 -5.08,-1.27; 2 -5.08,1.27; 3 -2.54,-1.27; 4 -2.54,1.27; 5 0,-1.27; 6 0,1.27; 7 2.54,-1.27; 8 2.54,1.27; 9 5.08,-1.27; 10 5.08,1.27

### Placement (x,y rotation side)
C1  53.98,51.44 90 top
C2  5.71,80.64 90 top
C3  41.91,51.44 90 top
C4  28.57,51.44 90 top
C5  15.88,51.44 90 top
C6  121.28,40.96 270 top
C7  127.95,22.23 270 top
C8  12.7,49.53 90 top
C9  58.42,67.31 0 bottom
C10  40.64,80.64 90 top
C11  25.4,67.31 0 bottom
C12  5.08,51.44 270 top
C13  69.22,31.75 90 top
C14  50.8,49.53 90 top
C15  38.1,49.53 90 top
C16  25.4,49.53 90 top
C17  93.34,21.59 0 top
C18  106.68,31.11 180 top
C19  84.45,47.62 90 bottom
C20  114.62,36.51 90 top
C21  88.9,47.62 270 bottom
C22  31.75,67.31 180 bottom
C23  64.14,67.31 180 bottom
C24  106.05,93.66 270 bottom
C26  76.83,31.11 90 top
E1  86.68,24.77 180 top
IC1  29.21,76.83 180 top
IC2  60.96,76.83 180 top
IC3  109.86,36.83 0 top
IC4  101.6,24.77 180 top
IC5  46.99,34.29 270 top
IC6  34.29,34.29 270 top
IC7  21.59,34.29 270 top
IC8  8.89,34.29 270 top
IC9  86.36,46.35 270 top
IC10  11.43,71.75 0 top
IC11  46.35,71.75 0 top
IC12  64.77,24.77 180 top
IC13  MIC5209  [SOT223']  117.79,31.43 270 top
QG1  113.67,52.39 180 top
R1  26.04,94.61 0 bottom
U$1  132.08,0 90 top
X1  100.97,88.27 0 top

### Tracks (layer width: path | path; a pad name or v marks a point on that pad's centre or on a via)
A1  (via drill 0.36)
  Top 0.305: IC1.25 v23.46,59.05 | IC2.25 v55.21,59.05 | IC9.2 v89.56,59.05
  Bottom 0.305: v23.46,59.05 v55.21,59.05 v89.56,59.05
A2  (via drill 0.36)
  Top 0.305: IC1.48 v34.96,69.22 | IC2.48 v66.71,69.22 | IC9.3 v88.76,69.22
  Bottom 0.305: v34.96,69.22 v66.71,69.22 v88.76,69.22
A3  (via drill 0.36)
  Top 0.305: IC1.23 v23.96,78.74 | IC2.23 v55.71,78.74 | IC9.14 77.61,48.76 76.83,49.53 v76.83,78.74
  Bottom 0.305: v23.96,78.74 v55.71,78.74 v76.83,78.74
A4  (via drill 0.36)
  Top 0.305: IC1.22 v24.46,92.71 | IC2.22 v56.21,92.71 | IC9.15 77.14,47.95 76.2,48.9 v76.2,92.71
  Bottom 0.305: v56.21,92.71 57.15,92.71 | v56.21,92.71 v24.46,92.71 | v76.2,92.71 v56.21,92.71
A5  (via drill 0.36)
  Top 0.305: IC11.19 v41.91,83.82 | IC1.21 v24.96,83.82 | IC2.21 v56.71,83.82
  Bottom 0.305: v56.71,83.82 v41.91,83.82 v24.96,83.82
A6  (via drill 0.36)
  Top 0.305: IC10.19 v6.99,89.53 | v25.46,89.53 IC1.20 | IC2.20 v57.21,89.53
  Bottom 0.305: v6.99,89.53 v25.46,89.53 v57.21,89.53
A7  (via drill 0.36)
  Top 0.305: IC10.18 v8.26,83.19 | v25.96,83.19 IC1.19 | IC2.19 v57.71,83.19
  Bottom 0.305: v8.26,83.19 v25.96,83.19 v57.71,83.19
A8  (via drill 0.36)
  Top 0.305: IC10.17 v9.53,90.17 | v26.46,90.17 IC1.18 | IC2.18 v58.21,90.17
  Bottom 0.305: v9.53,90.17 v26.46,90.17 v58.21,90.17
A9  (via drill 0.36)
  Top 0.305: IC10.16 v10.79,82.55 | v31.46,82.55 IC1.8 | IC2.8 v63.21,82.55
  Bottom 0.305: v10.79,82.55 v31.46,82.55 v63.21,82.55
A10  (via drill 0.36)
  Top 0.305: IC10.15 v12.06,90.81 | v31.96,90.81 IC1.7 | IC2.7 v63.71,90.81
  Bottom 0.305: v12.06,90.81 v31.96,90.81 v63.71,90.81
A11  (via drill 0.36)
  Top 0.305: IC10.14 v13.34,81.92 | v32.46,81.92 IC1.6 | IC2.6 v64.21,81.92
  Bottom 0.305: v13.34,81.92 v32.46,81.92 v64.21,81.92
A12  (via drill 0.36)
  Top 0.305: IC10.13 v14.61,91.44 | v32.96,91.44 IC1.5 | IC2.5 v64.71,91.44
  Bottom 0.305: v14.61,91.44 v32.96,91.44 v64.71,91.44
A13  (via drill 0.36)
  Top 0.305: IC10.12 v15.88,81.28 | v33.46,81.28 IC1.4 | IC2.4 v65.21,81.28
  Bottom 0.305: v15.88,81.28 v33.46,81.28 v65.21,81.28
A14  (via drill 0.36)
  Top 0.305: IC11.18 v43.18,93.98 | IC1.3 v33.96,93.98 | IC2.3 v65.71,93.98
  Bottom 0.305: v65.71,93.98 v43.18,93.98 v33.96,93.98
A15  (via drill 0.36)
  Top 0.305: IC11.17 v44.45,85.09 | IC1.2 v34.46,85.09 | IC2.2 v66.21,85.09
  Bottom 0.305: v34.46,85.09 v44.45,85.09 v66.21,85.09
A16  (via drill 0.36)
  Top 0.305: IC11.16 v45.72,87.63 | IC1.1 v34.96,87.63 | IC2.1 v66.71,87.63
  Bottom 0.305: v66.71,87.63 v45.72,87.63 v34.96,87.63
A17  (via drill 0.36)
  Top 0.305: IC11.15 v46.99,92.08 | IC1.24 23.46,92.08 v23.53,92.08 | IC2.24 55.21,92.08 v55.28,92.08
  Bottom 0.305: v23.53,92.08 v55.28,92.08 v46.99,92.08
A18  (via drill 0.36)
  Top 0.305: IC11.14 v48.26,84.45 | IC1.17 v26.96,84.45 | IC2.17 v58.71,84.45
  Bottom 0.305: v58.71,84.45 v48.26,84.45 v26.96,84.45
A19  (via drill 0.36)
  Top 0.305: IC11.13 v49.53,88.9 | IC1.16 v27.46,88.9 | IC2.16 v59.21,88.9
  Bottom 0.305: v59.21,88.9 v49.53,88.9 v27.46,88.9
A20  (via drill 0.36)
  Top 0.305: IC11.12 v50.8,88.27 | IC1.9 v30.96,88.27 | IC2.9 v62.71,88.27
  Bottom 0.305: v62.71,88.27 v50.8,88.27 v30.96,88.27
BBS7  (via drill 0.36)
  Top 0.305: IC4.9 v97.16,19.05
  Bottom 0.305: U$1.AP2 89.85,18.1 90.81,19.05 v97.16,19.05
BDAL0
  Bottom 0.305: U$1.AU2 77.15,22.54 76.2,23.5 52.7,23.5 IC5.12
BDAL1
  Bottom 0.305: U$1.AV2 73.98,21.27 72.39,22.86 IC5.11
BDAL2
  Bottom 0.305: U$1.BE2 45.4,23.18 IC5.9
BDAL3
  Bottom 0.305: U$1.BF2 42.23,12.38 41.91,12.7 41.91,26.67 IC5.8
BDAL4
  Bottom 0.305: U$1.BH2 39.05,13.65 39.37,13.97 39.37,24.13 IC6.12
BDAL5
  Bottom 0.305: U$1.BJ2 35.88,20.64 IC6.11
BDAL6
  Bottom 0.305: U$1.BK2 32.7,23.18 IC6.9
BDAL7
  Bottom 0.305: U$1.BL2 29.53,11.11 29.21,11.43 29.21,26.67 IC6.8
BDAL8
  Bottom 0.305: U$1.BM2 26.35,12.38 26.67,12.7 26.67,24.13 IC7.12
BDAL9
  Bottom 0.305: U$1.BN2 23.18,20.64 IC7.11
BDAL10
  Bottom 0.305: U$1.BP2 20,23.18 IC7.9
BDAL11
  Bottom 0.305: U$1.BR2 16.83,12.38 16.51,12.7 16.51,26.67 IC7.8
BDAL12
  Bottom 0.305: IC8.12 13.97,24.13 13.97,8.26 U$1.BS2
BDAL13
  Bottom 0.305: U$1.BT2 10.48,20.64 IC8.11
BDAL14
  Bottom 0.305: U$1.BU2 7.3,23.18 IC8.9
BDAL15
  Bottom 0.305: U$1.BV2 4.13,15.56 5.71,17.14 5.71,20.32 3.81,22.23 3.81,26.67 IC8.8
BDAL16  (via drill 0.36)
  Top 0.305: U$1.AC1 121.6,16.19 119.06,18.73 v119.06,27.62 | v64.14,27.62 IC12.5
  Bottom 0.305: v119.06,27.62 v64.14,27.62
BDAL17  (via drill 0.36)
  Top 0.305: U$1.AD1 v118.43,28.26 | v66.67,28.26 IC12.3
  Bottom 0.305: v118.43,28.26 v66.67,28.26
BDAL18
  Top 0.305: U$1.BC1 51.75,15.56 52.7,16.51 62.87,16.51 66.67,20.32 IC12.14
BDAL19
  Top 0.305: U$1.BD1 48.58,16.19 49.53,17.14 59.69,17.14 62.87,20.32 IC12.11
BDAL20
  Top 0.305: U$1.BE1 45.4,16.83 46.35,17.78 57.78,17.78 60.33,20.32 IC12.9
BDAL21
  Top 0.305: U$1.BF1 42.23,17.46 43.18,18.41 53.34,18.41 61.59,26.67 IC12.7
BDIN  (via drill 0.36)
  Top 0.305: v108.9,22.23 108.9,24.45 107.95,25.4 99.06,25.4 98.42,26.04 IC4.7
  Bottom 0.305: U$1.AH2 v108.9,22.23
BDOUT  (via drill 0.36)
  Top 0.305: v115.25,26.04 101.6,26.04 100.97,26.67 IC4.5
  Bottom 0.305: U$1.AE2 v115.25,26.04
BREF
  Top 0.305: U$1.AR1 87,8.26 86.68,8.26 E1.11
BRPLY  (via drill 0.36)
  Top 0.305: v84.14,26.99 E1.6
  Bottom 0.305: U$1.AF2 112.08,26.04 111.12,26.99 v84.14,26.99
BSYNC  (via drill 0.36)
  Top 0.305: IC4.14 v103.5,19.05
  Bottom 0.305: U$1.AJ2 105.73,18.1 104.78,19.05 v103.5,19.05
BWTBT  (via drill 0.36)
  Top 0.305: IC4.11 v99.69,18.41
  Bottom 0.305: U$1.AK2 102.55,17.46 101.6,18.41 v99.69,18.41
CE  (via drill 0.36)
  Top 0.305: IC1.12 v29.46,94.61 | IC2.12 v61.21,94.61
  Bottom 0.305: v61.21,94.61 v29.46,94.61 R1.1
CE0  (via drill 0.36)
  Top 0.305: IC1.26 v23.96,75.56 | IC9.19 75.89,44.76 74.93,45.72 v74.93,75.56
  Bottom 0.305: v23.96,75.56 v74.93,75.56
CE1  (via drill 0.36)
  Top 0.305: IC2.26 v55.71,76.2 | IC9.18 76.36,45.55 75.56,46.35 v75.56,76.2
  Bottom 0.305: v55.71,76.2 v75.56,76.2
CLK
  Top 0.305: IC9.37 103.81,44.76 106.05,46.99 QG1.8
DAL0  (via drill 0.36)
  Top 0.305: IC5.18 48.9,40.64 48.26,41.27 v48.26,58.42 | v25.46,58.42 IC1.29 | v57.21,58.42 IC2.29 | IC9.38 95.72,45.55 97.16,46.99 v97.16,58.42
  Bottom 0.305: v57.21,58.42 v25.46,58.42 | v48.26,58.42 v57.21,58.42 | v97.16,58.42 v57.21,58.42
DAL1  (via drill 0.36)
  Top 0.305: IC5.17 48.16,38.1 47.53,38.73 47.62,38.73 v47.62,57.78 | v26.46,57.78 IC1.31 | v58.21,57.78 IC2.31 | IC9.39 95.25,46.35 96.52,47.62 v96.52,57.78
  Bottom 0.305: v58.21,57.78 v26.46,57.78 | v47.62,57.78 v58.21,57.78 | v96.52,57.78 v58.21,57.78
DAL2  (via drill 0.36)
  Top 0.305: IC5.7 45.72,30.48 46.99,31.75 v46.99,57.15 | v27.46,57.15 IC1.33 | v59.21,57.15 IC2.33 | IC9.40 94.78,47.16 95.89,48.26 v95.89,57.15
  Bottom 0.305: v59.21,57.15 v27.46,57.15 | v46.99,57.15 v59.21,57.15 | v95.89,57.15 v59.21,57.15
DAL3  (via drill 0.36)
  Top 0.305: IC5.6 45.09,33.02 46.35,34.29 v46.35,56.52 | v28.46,56.52 IC1.35 | v60.21,56.52 IC2.35 | IC9.42 94.47,48.76 95.25,49.53 v95.25,56.52
  Bottom 0.305: v28.46,56.52 v46.35,56.52 v60.21,56.52 v95.25,56.52
DAL4  (via drill 0.36)
  Top 0.305: IC6.18 35.56,40.64 34.92,41.27 v34.92,55.88 | v87.16,55.88 IC9.5 | v29.96,55.88 IC1.38 | v61.71,55.88 IC2.38
  Bottom 0.305: v87.16,55.88 v61.71,55.88 v34.92,55.88 v29.96,55.88
DAL5  (via drill 0.36)
  Top 0.305: IC6.17 34.92,38.1 34.29,38.73 v34.29,59.69 | v44.45,59.69 IC11.4 | v30.96,59.69 IC1.40 | IC2.40 v62.71,59.69
  Bottom 0.305: v30.96,59.69 v34.29,59.69 v44.45,59.69 v62.71,59.69
DAL6  (via drill 0.36)
  Top 0.305: IC6.7 32.38,30.48 33.66,31.75 v33.66,60.33 | v41.91,60.33 IC11.2 | v31.96,60.33 IC1.42 | IC2.42 v63.71,60.33
  Bottom 0.305: v31.96,60.33 v33.66,60.33 v41.91,60.33 v63.71,60.33
DAL7  (via drill 0.36)
  Top 0.305: IC6.6 31.75,33.02 32.96,34.23 v32.96,60.96 IC1.44 | v43.18,60.96 IC11.3 | IC2.44 v64.71,60.96
  Bottom 0.305: v64.71,60.96 v43.18,60.96 v32.96,60.96
DAL8  (via drill 0.36)
  Top 0.305: IC7.18 22.23,40.64 21.59,41.27 v21.59,74.3 | v25.96,74.3 IC1.30 | IC10.9 v15.88,74.3 | IC2.30 v57.71,74.3
  Bottom 0.305: v15.88,74.3 v21.59,74.3 v25.96,74.3 v57.71,74.3
DAL9  (via drill 0.36)
  Top 0.305: IC10.8 v14.61,73.66 | v26.96,73.66 IC1.32 | IC7.17 21.59,38.1 20.95,38.73 v20.95,73.66 | IC2.32 v58.71,73.66
  Bottom 0.305: v14.61,73.66 v20.95,73.66 v26.96,73.66 v58.71,73.66
DAL10  (via drill 0.36)
  Top 0.305: IC7.7 19.05,30.48 20.32,31.75 v20.32,73.03 | IC10.7 v13.34,73.03 | v27.96,73.03 IC1.34 | IC2.34 v59.71,73.03
  Bottom 0.305: v13.34,73.03 v20.32,73.03 v27.96,73.03 v59.71,73.03
DAL11  (via drill 0.36)
  Top 0.305: IC7.6 19.05,33.02 19.68,33.66 v19.68,72.39 | v28.96,72.39 IC1.36 | v12.06,72.39 IC10.6 | IC2.36 v60.71,72.39
  Bottom 0.305: v12.06,72.39 v19.68,72.39 v28.96,72.39 v60.71,72.39
DAL12  (via drill 0.36)
  Top 0.305: IC8.18 10.79,42.55 v10.79,71.75 IC10.5 | v30.46,71.75 IC1.39 | IC2.39 v62.21,71.75
  Bottom 0.305: v10.79,71.75 v30.46,71.75 v62.21,71.75
DAL13  (via drill 0.36)
  Top 0.305: IC8.17 10.16,38.1 9.53,38.73 v9.53,71.12 IC10.4 | v31.46,71.12 IC1.41 | IC2.41 v63.21,71.12
  Bottom 0.305: v9.53,71.12 v31.46,71.12 v63.21,71.12
DAL14  (via drill 0.36)
  Top 0.305: IC8.7 7.62,30.48 8.26,31.11 v8.26,70.48 IC10.3 | v32.46,70.48 IC1.43 | IC2.43 v64.21,70.48
  Bottom 0.305: v8.26,70.48 v32.46,70.48 v64.21,70.48
DAL15  (via drill 0.36)
  Top 0.305: IC8.6 6.35,33.02 6.99,33.66 v6.99,69.85 IC10.2 | v33.46,69.85 IC1.45 | IC2.45 v65.21,69.85
  Bottom 0.305: v6.99,69.85 v33.46,69.85 v65.21,69.85
DAL16  (via drill 0.36)
  Top 0.305: v45.72,61.59 IC11.5 | v67.31,61.59 67.31,31.75 65.41,29.84 IC12.4
  Bottom 0.305: v67.31,61.59 v45.72,61.59
DAL17  (via drill 0.36)
  Top 0.305: v46.99,62.23 IC11.6 | v67.94,62.23 IC12.2
  Bottom 0.305: v67.94,62.23 v46.99,62.23
DAL18  (via drill 0.36)
  Top 0.305: v71.75,64.14 71.75,24.77 71.12,24.13 69.22,24.13 67.94,22.86 IC12.15 | IC11.9 v50.8,64.14
  Bottom 0.305: v71.75,64.14 v50.8,64.14
DAL19  (via drill 0.36)
  Top 0.305: v71.12,63.5 71.12,25.4 70.48,24.77 65.41,24.77 64.14,23.5 IC12.12 | IC11.8 v49.53,63.5
  Bottom 0.305: v71.12,63.5 v49.53,63.5
DAL20  (via drill 0.36)
  Top 0.305: v70.48,62.87 70.48,26.04 69.85,25.4 62.87,25.4 61.59,24.13 IC12.10 61.59,20.95 | IC11.7 v48.26,62.87
  Bottom 0.305: v70.48,62.87 v48.26,62.87
DAL21  (via drill 0.36)
  Top 0.305: IC9.22 v74.93,42.35 | v62.87,42.35 IC12.6
  Bottom 0.305: v74.93,42.35 v62.87,42.35
GND  (via drill 0.36)
  Top 0.305: IC2.27 56.21,66.04 | IC2.46 65.71,66.04 | IC1.27 24.46,66.04 | IC1.46 33.96,66.04
  Top 1.016: U$1.BT1 10.48,18.41 | U$1.BM1 26.35,19.37 | U$1.BJ1 35.88,19.05 | U$1.AT1 80.33,17.46 | U$1.AM1 96.2,17.14 | U$1.AJ1 105.73,17.46
  Bottom 0.61: C24.2 X1.10
  Bottom 0.813: C21.2 v88.9,45.72 | C19.2 v84.45,49.53 | C22.2 v35.88,67.31 | C23.2 v67.94,67.31 | C11.2 v22.54,67.31 | C9.2 v54.29,67.31
  Bottom 1.016: U$1.AC2 v121.6,19.37
  Bottom 1.27: U$1.BC2 v51.75,19.37 v51.75,20.32
  other vias: 121.6,18.41 121.6,17.46
  pour Top (isolate 0.254): 0.64,99.69 131.44,99.69 131.44,16.51 0.64,16.51
LB  (via drill 0.36)
  Top 0.305: IC1.15 27.96,85.72 27.94,85.72 v27.94,80.01 | IC2.15 v59.71,80.01 | IC9.21 74.95,43.16 74.3,43.81 74.3,80 v74.28,80.01
  Bottom 0.305: v27.94,80.01 v59.71,80.01 v74.28,80.01
LE  (via drill 0.36)
  Top 0.305: IC9.12 79.19,50.35 78.11,51.44 v78.11,79.38 | IC10.11 v17.14,79.38 | IC11.11 v52.07,79.38
  Bottom 0.305: v17.14,79.38 v52.07,79.38 v78.11,79.38
N$1
  Bottom 0.305: U$1.AS2 83.5,15.56 83.82,15.88 86.36,15.88 86.68,15.56 U$1.AR2
N$2
  Bottom 0.305: U$1.AN2 93.03,15.56 93.34,15.88 95.89,15.88 96.2,15.56 U$1.AM2
OE  (via drill 0.36)
  Top 0.305: IC1.28 v24.96,74.93 | IC2.28 v56.71,74.93 | IC9.10 v83.16,74.93
  Bottom 0.305: v24.96,74.93 v56.71,74.93 v83.16,74.93
RBS7
  Top 0.305: IC9.30 87.96,35.87 92.08,31.75 92.08,24.13 92.71,23.5 97.79,23.5 98.42,22.86 IC4.10
RDIN
  Top 0.305: IC9.34 98.61,42.35 99.69,41.27 IC4.6
RDOUT
  Top 0.305: IC9.35 101.62,43.16 102.23,42.55 IC4.4
REC  (via drill 0.36)
  Top 0.305: v83.96,39.37 IC9.25
  Bottom 0.305: IC8.4 9.53,38.1 10.79,39.37 14.61,39.37 15.88,38.1 IC7.4 22.86,38.1 24.13,39.37 27.3,39.37 28.57,38.1 IC6.4 34.92,38.1 36.2,39.37 40.01,39.37 41.27,38.1 IC5.4 46.35,38.1 47.62,39.37 v83.96,39.37
RSYNC
  Top 0.305: IC9.33 90.36,36.01 93.34,33.02 93.34,25.4 93.98,24.77 104.14,24.77 104.78,24.13 IC4.15
RWTBT
  Top 0.305: IC9.31 88.76,36.34 92.71,32.38 92.71,24.77 93.34,24.13 100.33,24.13 100.97,23.5 IC4.12
TCK  (via drill 0.36)
  Top 0.305: IC9.26 v84.76,44.45 | v97.79,46.99 97.79,85.09 X1.1
  Bottom 0.305: v84.76,44.45 95.25,44.45 v97.79,46.99
TDI  (via drill 0.36)
  Top 0.305: IC9.1 v90.36,84.45
  Bottom 0.305: v90.36,84.45 103.5,84.45 X1.9
TDO  (via drill 0.36)
  Top 0.305: IC9.32 v89.56,43.81 | v98.42,46.35 X1.3
  Bottom 0.305: v89.56,43.81 95.89,43.81 v98.42,46.35
TMS  (via drill 0.36)
  Top 0.305: IC9.7 v85.56,85.09
  Bottom 0.305: v85.56,85.09 99.06,85.09 X1.5
TREF
  Top 0.305: IC9.28 86.36,36.2 91.44,31.11 91.44,24.13 90.81,23.5 90.17,23.5 89.22,22.54 E1.13 E1.12
TRPLY
  Top 0.305: IC9.27 85.56,28.41 85.41,28.26 E1.5 E1.4
UB  (via drill 0.36)
  Top 0.305: IC1.14 v28.46,93.34 | IC2.14 v60.21,93.34 | v77.47,93.34 77.47,50.8 78.72,49.55 IC9.13
  Bottom 0.305: v28.46,93.34 v60.21,93.34 v77.47,93.34
VCC  (via drill 0.36)
  Top 0.305: IC9.29 v87.16,41.91 | v29.21,65.72 29.46,65.97 IC1.37 29.46,68.19 v29.84,68.58 | v60.96,65.72 61.21,65.97 IC2.37 61.21,68.19 v61.59,68.58 | IC9.9 v83.96,50.8 | IC9.17 v81.92,46.35 | IC9.41 v90.81,47.95 | IC1.47 34.46,68.41 v34.29,68.58 | IC2.47 66.21,68.41 v66.04,68.58 | IC13.1 114.69,34.29 114.69,34.61 v114.3,34.61 v115.25,34.61
  Top 0.61: C17.1 v91.44,21.59 90.49,21.59 E1.14 | IC10.20 v5.71,78.11 C2.1 | IC11.20 v40.64,78.11 C10.1 | C12.+ v5.08,54.61
  Top 1.016: C7.+ v127.95,25.08 | U$1.BV1 v4.13,19.68 | IC5.20 C14.1 53.98,48.58 C1.+ | IC6.20 C15.1 41.91,48.58 C3.+ | IC7.20 C16.1 28.57,48.58 C4.+ | IC8.20 C8.1 15.88,48.58 C5.+ | IC3.3 114.69,33.68 114.69,34.29
  Top 1.27: C20.1 114.62,33.74 IC13.1
  Top 1.422: C6.+ QG1.14
  Bottom 1.016: U$1.AA2 127.95,17.14 | U$1.BA2 58.1,17.46
  other vias: 127,25.08 128.91,25.08 4.13,18.73 4.13,17.78 6.03,54.61 4.13,54.61
  pour Bottom (isolate 0.254): 0.64,99.69 131.44,99.69 131.44,16.51 0.64,16.51 0.64,99.06
VDD  (via drill 0.36)
  Top 0.61: C13.1 v69.22,29.21 IC12.1 | IC4.1 v106.05,29.21
  Top 0.813: C26.+ v76.83,29.21 | IC13.3 114.69,29.21 109.86,29.21 | 109.86,29.21 v107.63,29.21 | v107.63,29.21 v106.05,29.21 | IC3.2 109.86,33.68 109.86,29.21 | v107.63,29.21 C18.1
  Bottom 0.61: v76.83,29.21 v77.47,29.21
  Bottom 0.813: v69.22,29.21 v76.2,29.21 v76.83,29.21 | v107.63,29.21 v106.05,29.21 v77.47,29.21 84.45,29.21
WE  (via drill 0.36)
  Top 0.305: IC1.11 v29.96,80.64 | IC9.11 v82.36,80.64 | IC2.11 v61.71,80.64
  Bottom 0.305: v29.96,80.64 v61.71,80.64 v82.36,80.64
XMIT  (via drill 0.36)
  Top 0.305: v82.36,36.83 IC9.23
  Bottom 0.305: IC8.5 9.53,35.56 10.79,36.83 14.61,36.83 15.88,35.56 IC7.5 22.86,35.56 24.13,36.83 27.3,36.83 28.57,35.56 IC6.5 34.92,35.56 36.2,36.83 40.01,36.83 41.27,35.56 IC5.5 46.35,35.56 47.62,36.83 v82.36,36.83

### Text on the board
tDocu: 4Mbyte Memory / Peter Schranz / April 2019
